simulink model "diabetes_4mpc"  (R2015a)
settings: Solver=ode45  StartTime=0.0  StopTime=24  RelTol=1e-3
StopFcn:
  | plot_results
libraries: simulink x1

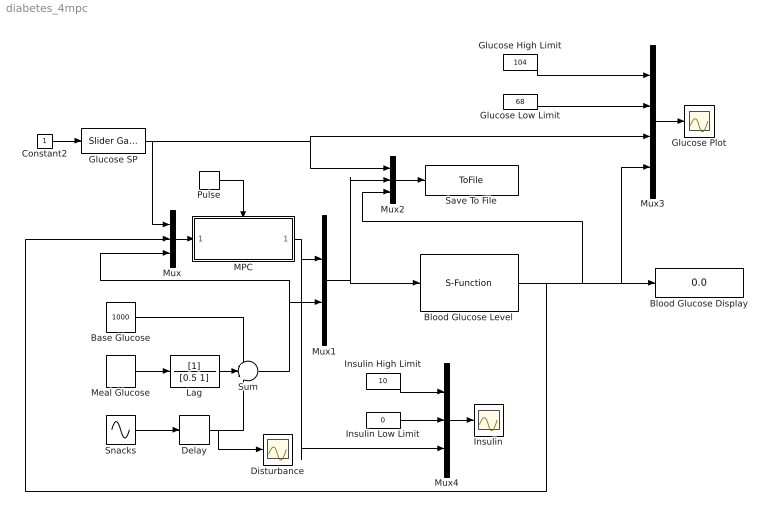
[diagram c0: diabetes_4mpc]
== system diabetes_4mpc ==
  Base Glucose : Constant  Value=1000
  Blood Glucose Display : Display
  Blood Glucose Level : S-Function  FunctionName=diabetic
  Constant2 : Constant
  Delay : TransportDelay  DelayTime=8
  Disturbance : Scope
  Glucose High Limit : Constant  Value=104
  Glucose Low Limit : Constant  Value=68
  Glucose Plot : Scope
  Glucose SP : simulink/Math Operations/Slider Gain  low=50  gain=80  high=120
  Insulin : Scope
  Insulin High Limit : Constant  Value=10
  Insulin Low Limit : Constant  Value=0
  Lag : TransferFcn  Denominator=[0.5 1]
  MPC : Subsystem  TreatAsAtomicUnit=on
  Meal Glucose : DiscretePulseGenerator  PulseType=Time based  Amplitude=500  Period=6  PulseWidth=10  PhaseDelay=7
  Mux : Mux  Inputs=3
  Mux1 : Mux  Inputs=2
  Mux2 : Mux  Inputs=3
  Mux3 : Mux
  Mux4 : Mux  Inputs=3
  Pulse : DiscretePulseGenerator  PulseType=Time based  Period=0.2  PulseWidth=5
  Save To File : ToFile  Filename=data.mat  MatrixName=diabetic  SampleTime=0.05
  Snacks : Sin  Amplitude=200  Frequency=0.5  SampleTime=0
  Sum : Sum  Inputs=+++
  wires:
  Mux2/1 -> Save To File/1
  Mux1/1 -> Mux2/2, Blood Glucose Level/1
  Constant2/1 -> Glucose SP/1
  Glucose SP/1 -> Mux/1, Mux3/3, Mux2/1
  Blood Glucose Level/1 -> Mux/2, Mux3/4, Blood Glucose Display/1, Mux2/3
  Glucose High Limit/1 -> Mux3/1
  Glucose Low Limit/1 -> Mux3/2
  Mux3/1 -> Glucose Plot/1
  MPC/1(Out1) -> Mux4/3, Mux1/1
  Base Glucose/1 -> Sum/1
  Snacks/1 -> Delay/1
  Delay/1 -> Disturbance/1, Sum/3
  Meal Glucose/1 -> Lag/1
  Sum/1 -> Mux1/2, Mux/3
  Lag/1 -> Sum/2
  Insulin High Limit/1 -> Mux4/1
  Insulin Low Limit/1 -> Mux4/2
  Mux4/1 -> Insulin/1
  Mux/1 -> MPC/1(In1)
  Pulse/1 -> MPC/Trigger

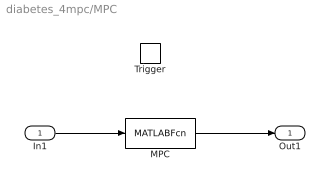
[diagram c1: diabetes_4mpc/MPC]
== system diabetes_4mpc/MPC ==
  In1 : Inport
  Trigger : TriggerPort
  MPC : MATLABFcn  MATLABFcn=mpc
  Out1 : Outport
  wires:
  In1/1 -> MPC/1
  MPC/1 -> Out1/1
